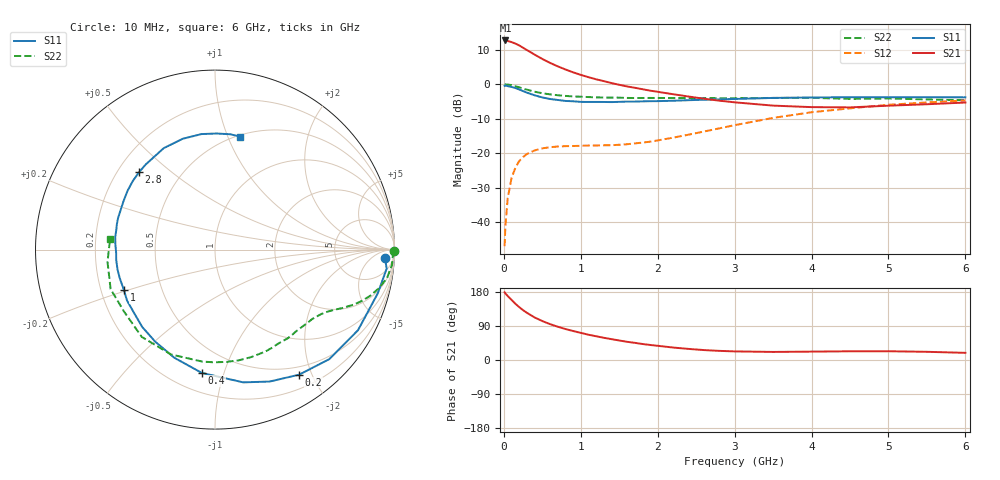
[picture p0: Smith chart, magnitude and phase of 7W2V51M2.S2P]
! Infineon Technologies  Discrete & RF Semiconductors
! BFS17W
! Si NPN RF Bipolar Junction Transistor in SOT323
! VCE = 2.5 V  IC = 1.2 mA
! Common Emitter S-Parameters:  August  1999
# GHz  S  MA  R  50
!  f  S11  S21  S12  S22
! GHz  MAG  ANG  MAG  ANG  MAG  ANG  MAG  ANG
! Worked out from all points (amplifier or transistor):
!   36 points, 10 MHz to 6 GHz, reference 50 ohm
!   highest |S21| = 12.7 dB at 20 MHz (marker M1)
!   |S21| within 3 dB of that: start of sweep to 316.7 MHz
!   unconditionally stable (mu >= 1): 963.5 MHz to end of sweep
!   at 250 MHz: K = 0.29, MSG = 15.8 dB, |S12| = -21.1 dB
!   at 1.4 GHz: K = 1.31, MAG = 5.7 dB, |S12| = -17.7 dB
!   at 6 GHz: K = 1.11, MAG = -2.3 dB, |S12| = -4.7 dB
!   S11 on the Smith chart (normalised r, x): 10 MHz: 20, -19; 200 MHz: 0.38, -1.81; 400 MHz: 0.32, -0.85; 1 GHz: 0.30, -0.19; 2.8 GHz: 0.29, +0.39; 6 GHz: 0.51, +1.11
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0.01  0.9482 -2.9  4.264 178.6  0.0045 86.5  0.9996 -0.5
0.02  0.9624 -6.3  4.311 175.7  0.0087 88.2  0.9917 -1.9
0.05  0.9392 -15.0  4.233 168.9  0.0221 82.5  0.9898 -4.9
0.1  0.9147 -29.4  4.085 158.7  0.0438 73.8  0.9716 -9.4
0.15  0.882 -43.8  3.881 148.4  0.0615 65.1  0.9367 -13.4
0.2  0.8397 -56.1  3.653 139.5  0.0771 59.5  0.9018 -16.6
0.25  0.7957 -67.5  3.379 131.5  0.0881 53.1  0.8658 -19.3
0.3  0.7562 -78.0  3.13 124.5  0.0976 49.1  0.8353 -21.4
0.4  0.691 -96.1  2.69 112.3  0.1099 42.0  0.7798 -24.7
0.5  0.6438 -110.6  2.326 102.8  0.1177 37.6  0.741 -27.0
0.6  0.6116 -123.0  2.041 94.7  0.1223 34.3  0.7135 -29.1
0.7  0.5919 -133.2  1.818 87.9  0.1251 32.9  0.6933 -31.1
0.8  0.5727 -141.9  1.638 81.8  0.1267 31.7  0.6779 -33.4
1  0.5552 -156.2  1.367 71.6  0.1282 31.9  0.6597 -37.5
1.1  0.554 -163.1  1.266 66.7  0.1293 32.9  0.652 -40.2
1.6  0.5604 172.7  0.93 48.1  0.135 41.2  0.6337 -53.6
2.2  0.5764 152.3  0.717 32.9  0.1682 54.5  0.6319 -71.5
2.8  0.6041 134.5  0.578 24.1  0.2293 60.2  0.628 -90.5
3.5  0.6333 116.8  0.49 21.3  0.3253 58.1  0.6334 -112.7
4.5  0.648 96.6  0.462 23.0  0.4473 46.2  0.6133 -145.7
5.5  0.6481 82.6  0.513 21.6  0.5444 33.7  0.6028 -173.5
6  0.6454 77.4  0.543 18.9  0.5822 27.7  0.5876 174.3
